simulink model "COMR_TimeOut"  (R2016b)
settings: Solver=FixedStepDiscrete  StartTime=0.0  StopTime=10.0  FixedStep=0.01  RelTol=1e-3  EnableMultiTasking=on
undefined symbols (not defined in the file or in its folder): bin2dec, COMR_cntObcTmtDiag_CW, COMR_cntVcu2A3TmtDiag_CW, COMR_flgTmtCAB_C, COMR_numPackVcuMsg_C, COMR_tiBusoffDiagEna_C, COMR_tiCabMsgTmt_C, COMR_tiCSCMsgTmt_C, COMR_tiGWMsg050Tmt_C, COMR_tiGWMsgTmt_C, COMR_tiHv638MsgTmt_C, COMR_tiMcuMsgTmt_C, COMR_tiObcMsgTmt_C, COMR_tiPackVcuMsgTmt_C, COMR_tiPwrupDiagEna_C, COMR_tiTmtBase_C, COMR_tiVcuMsgTmt_C, COMR_UAESFltDiagDisbl_C
libraries: simulink x167
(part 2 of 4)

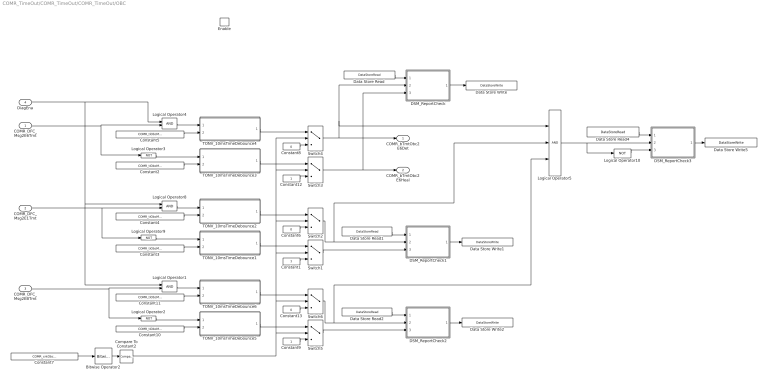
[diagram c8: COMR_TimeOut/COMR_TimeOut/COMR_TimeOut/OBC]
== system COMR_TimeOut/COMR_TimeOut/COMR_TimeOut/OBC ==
  COMR_DFC_Msg2E6Tmt : Inport
  COMR_DFC_Msg2E1Tmt : Inport  Port=2
  COMR_DFC_Msg2EBTmt : Inport  Port=3
  DiagEna : Inport  Port=4
  Enable : EnablePort
  Bitwise Operator2 : simulink/Logic and Bit Operations/Bitwise Operator  logicop=AND  UseBitMask=on  BitMask=bin2dec('00010000')  BitMaskRealWorld=Stored Integer
  Compare To Constant2 : simulink/Logic and Bit Operations/Compare To Constant  relop===  const=16  OutDataTypeStr=boolean
  Constant1 : Constant  OutDataTypeStr=boolean
  Constant{2..5,10..11} (6 alike) : Constant  Value=COMR_tiObcMsgTmt_C
  Constant12 : Constant  OutDataTypeStr=boolean
  Constant13 : Constant  Value=0  OutDataTypeStr=boolean
  Constant6 : Constant  Value=0  OutDataTypeStr=boolean
  Constant7 : Constant  Value=COMR_cntObcTmtDiag_CW
  Constant8 : Constant  Value=0  OutDataTypeStr=boolean
  Constant9 : Constant  OutDataTypeStr=boolean
  DSM_ReportCheck : Subsystem  TreatAsAtomicUnit=on  RTWFcnName=DSM_ReportCheck  RTWFileName=SrvLib
  DSM_ReportCheck1 : Subsystem  TreatAsAtomicUnit=on  RTWFcnName=DSM_ReportCheck  RTWFileName=SrvLib
  DSM_ReportCheck2 : Subsystem  TreatAsAtomicUnit=on  RTWFcnName=DSM_ReportCheck  RTWFileName=SrvLib
  DSM_ReportCheck3 : Subsystem  TreatAsAtomicUnit=on  RTWFcnName=DSM_ReportCheck  RTWFileName=SrvLib
  Data Store Read : DataStoreRead  DataStoreName=DFC_Msg2E6Tmt
  Data Store Read1 : DataStoreRead  DataStoreName=DFC_Msg2E1Tmt
  Data Store Read2 : DataStoreRead  DataStoreName=DFC_Msg2EBTmt
  Data Store Read4 : DataStoreRead  DataStoreName=DFC_ObcTmt
  Data Store Write : DataStoreWrite  DataStoreName=DFC_Msg2E6Tmt
  Data Store Write1 : DataStoreWrite  DataStoreName=DFC_Msg2E1Tmt
  Data Store Write2 : DataStoreWrite  DataStoreName=DFC_Msg2EBTmt
  Data Store Write5 : DataStoreWrite  DataStoreName=DFC_ObcTmt
  Logical Operator1 : Logic  AllPortsSameDT=off  OutDataTypeStr=boolean
  Logical Operator{2..3,9..10} (4 alike) : Logic  Operator=NOT  AllPortsSameDT=off  OutDataTypeStr=boolean
  Logical Operator4 : Logic  AllPortsSameDT=off  OutDataTypeStr=boolean
  Logical Operator5 : Logic  Inputs=3  AllPortsSameDT=off  OutDataTypeStr=boolean
  Logical Operator8 : Logic  AllPortsSameDT=off  OutDataTypeStr=boolean
  Switch{1..6} (6 alike) : Switch  Criteria=u2 > Threshold
  TONV_10msTimeDebounce1 : Subsystem  TreatAsAtomicUnit=on  RTWFcnName=TONV_10msTimeDebounce  RTWFileName=SrvLib
  TONV_10msTimeDebounce2 : Subsystem  TreatAsAtomicUnit=on  RTWFcnName=TONV_10msTimeDebounce  RTWFileName=SrvLib
  TONV_10msTimeDebounce3 : Subsystem  TreatAsAtomicUnit=on  RTWFcnName=TONV_10msTimeDebounce  RTWFileName=SrvLib
  TONV_10msTimeDebounce4 : Subsystem  TreatAsAtomicUnit=on  RTWFcnName=TONV_10msTimeDebounce  RTWFileName=SrvLib
  TONV_10msTimeDebounce5 : Subsystem  TreatAsAtomicUnit=on  RTWFcnName=TONV_10msTimeDebounce  RTWFileName=SrvLib
  TONV_10msTimeDebounce6 : Subsystem  TreatAsAtomicUnit=on  RTWFcnName=TONV_10msTimeDebounce  RTWFileName=SrvLib
  COMR_bTmtObc2E6Det : Outport  OutputWhenDisabled=reset  InitialOutput=[0]
  COMR_bTmtObc2E6Heal : Outport  Port=2  OutputWhenDisabled=reset  InitialOutput=[0]
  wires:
  Constant5/1 -> TONV_10msTimeDebounce4/2(T)
  DSM_ReportCheck/1(Dfc_id) -> Data Store Write/1
  Constant2/1 -> TONV_10msTimeDebounce3/2(T)
  Constant8/1 -> Switch4/3
  Constant12/1 -> Switch3/3
  TONV_10msTimeDebounce4/1(y) -> Switch4/1
  TONV_10msTimeDebounce3/1(y) -> Switch3/1
  Switch3/1 -> DSM_ReportCheck/3(Heal), COMR_bTmtObc2E6Heal/1
  Data Store Read/1 -> DSM_ReportCheck/1(Dfc_id_nv)
  Logical Operator3/1 -> TONV_10msTimeDebounce3/1(u)
  Switch4/1 -> DSM_ReportCheck/2(Err), Logical Operator5/1, COMR_bTmtObc2E6Det/1
  COMR_DFC_Msg2E6Tmt/1 -> Logical Operator3/1, Logical Operator4/2
  Logical Operator4/1 -> TONV_10msTimeDebounce4/1(u)
  Constant4/1 -> TONV_10msTimeDebounce2/2(T)
  DSM_ReportCheck1/1(Dfc_id) -> Data Store Write1/1
  Constant3/1 -> TONV_10msTimeDebounce1/2(T)
  Compare To Constant2/1 -> Switch5/2, Switch6/2, Switch3/2, Switch4/2, Switch2/2, Switch1/2
  Constant7/1 -> Bitwise Operator2/1
  Bitwise Operator2/1 -> Compare To Constant2/1
  Constant6/1 -> Switch2/3
  Constant1/1 -> Switch1/3
  TONV_10msTimeDebounce2/1(y) -> Switch2/1
  TONV_10msTimeDebounce1/1(y) -> Switch1/1
  Switch1/1 -> DSM_ReportCheck1/3(Heal)
  Data Store Read1/1 -> DSM_ReportCheck1/1(Dfc_id_nv)
  Switch2/1 -> DSM_ReportCheck1/2(Err), Logical Operator5/2
  COMR_DFC_Msg2E1Tmt/1 -> Logical Operator9/1, Logical Operator8/2
  Logical Operator8/1 -> TONV_10msTimeDebounce2/1(u)
  Logical Operator9/1 -> TONV_10msTimeDebounce1/1(u)
  DiagEna/1 -> Logical Operator1/1, Logical Operator8/1, Logical Operator4/1
  Constant11/1 -> TONV_10msTimeDebounce6/2(T)
  DSM_ReportCheck2/1(Dfc_id) -> Data Store Write2/1
  Constant10/1 -> TONV_10msTimeDebounce5/2(T)
  Constant13/1 -> Switch6/3
  Constant9/1 -> Switch5/3
  TONV_10msTimeDebounce6/1(y) -> Switch6/1
  TONV_10msTimeDebounce5/1(y) -> Switch5/1
  Switch5/1 -> DSM_ReportCheck2/3(Heal)
  Data Store Read2/1 -> DSM_ReportCheck2/1(Dfc_id_nv)
  Switch6/1 -> DSM_ReportCheck2/2(Err), Logical Operator5/3
  COMR_DFC_Msg2EBTmt/1 -> Logical Operator2/1, Logical Operator1/2
  Logical Operator1/1 -> TONV_10msTimeDebounce6/1(u)
  Logical Operator2/1 -> TONV_10msTimeDebounce5/1(u)
  Data Store Read4/1 -> DSM_ReportCheck3/1(Dfc_id_nv)
  DSM_ReportCheck3/1(Dfc_id) -> Data Store Write5/1
  Logical Operator5/1 -> DSM_ReportCheck3/2(Err), Logical Operator10/1
  Logical Operator10/1 -> DSM_ReportCheck3/3(Heal)

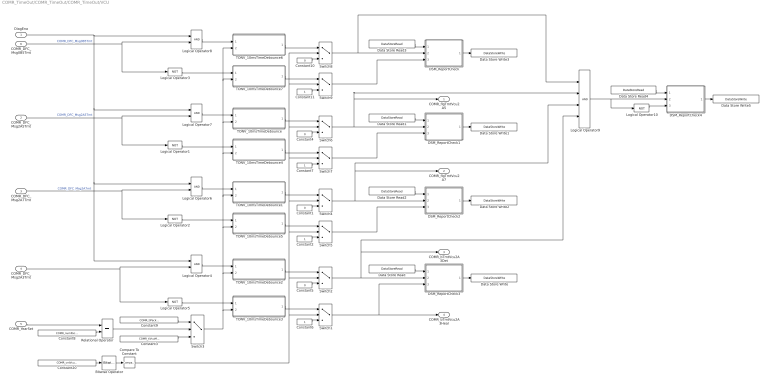
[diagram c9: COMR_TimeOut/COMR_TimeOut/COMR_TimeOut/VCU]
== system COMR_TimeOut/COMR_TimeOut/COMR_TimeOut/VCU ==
  DiagEna : Inport
  COMR_DFC_Msg2A5Tmt : Inport  Port=2
  COMR_DFC_Msg2A7Tmt : Inport  Port=3
  COMR_DFC_Msg2A3Tmt : Inport  Port=4
  COMR_YearSet : Inport  Port=5
  COMR_DFC_Msg0B5Tmt : Inport  Port=6
  Bitwise Operator : simulink/Logic and Bit Operations/Bitwise Operator  logicop=AND  UseBitMask=on  BitMask=bin2dec('00010000')  BitMaskRealWorld=Stored Integer
  Compare To Constant : simulink/Logic and Bit Operations/Compare To Constant  relop===  const=16  OutDataTypeStr=boolean
  Constant{1,4..5,10} (4 alike) : Constant  Value=0  OutDataTypeStr=boolean
  Constant{2,6..7,11} (4 alike) : Constant  OutDataTypeStr=boolean
  Constant20 : Constant  Value=COMR_cntVcu2A3TmtDiag_CW
  Constant3 : Constant  Value=COMR_tiVcuMsgTmt_C
  Constant8 : Constant  Value=COMR_numPackVcuMsg_C  OutDataTypeStr=uint16
  Constant9 : Constant  Value=COMR_tiPackVcuMsgTmt_C
  DSM_ReportCheck : Subsystem  TreatAsAtomicUnit=on  RTWFcnName=DSM_ReportCheck  RTWFileName=SrvLib
  DSM_ReportCheck1 : Subsystem  TreatAsAtomicUnit=on  RTWFcnName=DSM_ReportCheck  RTWFileName=SrvLib
  DSM_ReportCheck2 : Subsystem  TreatAsAtomicUnit=on  RTWFcnName=DSM_ReportCheck  RTWFileName=SrvLib
  DSM_ReportCheck3 : Subsystem  TreatAsAtomicUnit=on  RTWFcnName=DSM_ReportCheck  RTWFileName=SrvLib
  DSM_ReportCheck4 : Subsystem  TreatAsAtomicUnit=on  RTWFcnName=DSM_ReportCheck  RTWFileName=SrvLib
  Data Store Read : DataStoreRead  DataStoreName=DFC_Msg2A3Tmt
  Data Store Read1 : DataStoreRead  DataStoreName=DFC_Msg2A5Tmt
  Data Store Read2 : DataStoreRead  DataStoreName=DFC_Msg2A7Tmt
  Data Store Read3 : DataStoreRead  DataStoreName=DFC_Msg0B5Tmt
  Data Store Read4 : DataStoreRead  DataStoreName=DFC_VcuTmt
  Data Store Write : DataStoreWrite  DataStoreName=DFC_Msg2A3Tmt
  Data Store Write1 : DataStoreWrite  DataStoreName=DFC_Msg2A5Tmt
  Data Store Write2 : DataStoreWrite  DataStoreName=DFC_Msg2A7Tmt
  Data Store Write3 : DataStoreWrite  DataStoreName=DFC_Msg0B5Tmt
  Data Store Write5 : DataStoreWrite  DataStoreName=DFC_VcuTmt
  Logical Operator{1..3,5,10} (5 alike) : Logic  Operator=NOT  AllPortsSameDT=off  OutDataTypeStr=boolean
  Logical Operator{4,6..8} (4 alike) : Logic  AllPortsSameDT=off  OutDataTypeStr=boolean
  Logical Operator9 : Logic  Inputs=4  AllPortsSameDT=off  OutDataTypeStr=boolean
  Relational Operator : RelationalOperator  Operator===  OutDataTypeStr=boolean  RndMeth=Simplest
  Switch{1..2,4..9} (8 alike) : Switch  Criteria=u2 > Threshold
  Switch3 : Switch  Criteria=u2 ~= 0
  TONV_10msTimeDebounce : Subsystem  TreatAsAtomicUnit=on  RTWFcnName=TONV_10msTimeDebounce  RTWFileName=SrvLib
  TONV_10msTimeDebounce1 : Subsystem  TreatAsAtomicUnit=on  RTWFcnName=TONV_10msTimeDebounce  RTWFileName=SrvLib
  TONV_10msTimeDebounce2 : Subsystem  TreatAsAtomicUnit=on  RTWFcnName=TONV_10msTimeDebounce  RTWFileName=SrvLib
  TONV_10msTimeDebounce3 : Subsystem  TreatAsAtomicUnit=on  RTWFcnName=TONV_10msTimeDebounce  RTWFileName=SrvLib
  TONV_10msTimeDebounce4 : Subsystem  TreatAsAtomicUnit=on  RTWFcnName=TONV_10msTimeDebounce  RTWFileName=SrvLib
  TONV_10msTimeDebounce5 : Subsystem  TreatAsAtomicUnit=on  RTWFcnName=TONV_10msTimeDebounce  RTWFileName=SrvLib
  TONV_10msTimeDebounce6 : Subsystem  TreatAsAtomicUnit=on  RTWFcnName=TONV_10msTimeDebounce  RTWFileName=SrvLib
  TONV_10msTimeDebounce7 : Subsystem  TreatAsAtomicUnit=on  RTWFcnName=TONV_10msTimeDebounce  RTWFileName=SrvLib
  COMR_flgTmtVcu2A5 : Outport
  COMR_flgTmtVcu2A7 : Outport  Port=2
  COMR_bTmtVcu2A3Det : Outport  Port=3  OutputWhenDisabled=reset  InitialOutput=[0]
  COMR_bTmtVcu2A3Heal : Outport  Port=4  OutputWhenDisabled=reset  InitialOutput=[0]
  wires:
  COMR_DFC_Msg2A5Tmt/1 -> Logical Operator7/2, Logical Operator1/1  "COMR_DFC_Msg2A5Tmt"
  COMR_DFC_Msg2A7Tmt/1 -> Logical Operator6/2, Logical Operator2/1  "COMR_DFC_Msg2A7mt"
  Constant3/1 -> Switch3/3
  TONV_10msTimeDebounce2/1(y) -> Switch2/1
  Constant20/1 -> Bitwise Operator/1
  Bitwise Operator/1 -> Compare To Constant/1
  Constant5/1 -> Switch2/3
  Constant6/1 -> Switch1/3
  TONV_10msTimeDebounce3/1(y) -> Switch1/1
  Switch2/1 -> DSM_ReportCheck3/2(Err), Logical Operator9/4, COMR_bTmtVcu2A3Det/1
  Switch1/1 -> DSM_ReportCheck3/3(Heal), COMR_bTmtVcu2A3Heal/1
  DSM_ReportCheck3/1(Dfc_id) -> Data Store Write/1
  Data Store Read/1 -> DSM_ReportCheck3/1(Dfc_id_nv)
  COMR_DFC_Msg2A3Tmt/1 -> Logical Operator4/2, Logical Operator5/1
  Logical Operator4/1 -> TONV_10msTimeDebounce2/1(u)
  DiagEna/1 -> Logical Operator8/1, Logical Operator7/1, Logical Operator4/1, Logical Operator6/1
  COMR_YearSet/1 -> Relational Operator/1
  Relational Operator/1 -> Switch3/2
  Constant8/1 -> Relational Operator/2
  Constant9/1 -> Switch3/1
  Logical Operator5/1 -> TONV_10msTimeDebounce3/1(u)
  Data Store Read1/1 -> DSM_ReportCheck1/1(Dfc_id_nv)
  Switch6/1 -> DSM_ReportCheck1/2(Err), Logical Operator9/2, COMR_flgTmtVcu2A5/1
  DSM_ReportCheck1/1(Dfc_id) -> Data Store Write1/1
  Logical Operator1/1 -> TONV_10msTimeDebounce4/1(u)
  Switch7/1 -> DSM_ReportCheck1/3(Heal)
  Switch3/1 -> TONV_10msTimeDebounce3/2(T), TONV_10msTimeDebounce2/2(T), TONV_10msTimeDebounce6/2(T), TONV_10msTimeDebounce7/2(T), TONV_10msTimeDebounce/2(T), TONV_10msTimeDebounce4/2(T), TONV_10msTimeDebounce1/2(T), TONV_10msTimeDebounce5/2(T)
  Logical Operator2/1 -> TONV_10msTimeDebounce5/1(u)
  Data Store Read2/1 -> DSM_ReportCheck2/1(Dfc_id_nv)
  Switch4/1 -> DSM_ReportCheck2/2(Err), COMR_flgTmtVcu2A7/1, Logical Operator9/3
  DSM_ReportCheck2/1(Dfc_id) -> Data Store Write2/1
  COMR_DFC_Msg0B5Tmt/1 -> Logical Operator8/2, Logical Operator3/1  "COMR_DFC_Msg0B5Tmt"
  Data Store Read3/1 -> DSM_ReportCheck/1(Dfc_id_nv)
  Switch8/1 -> DSM_ReportCheck/2(Err), Logical Operator9/1
  DSM_ReportCheck/1(Dfc_id) -> Data Store Write3/1
  Logical Operator3/1 -> TONV_10msTimeDebounce7/1(u)
  Switch9/1 -> DSM_ReportCheck/3(Heal)
  TONV_10msTimeDebounce1/1(y) -> Switch4/1
  Constant1/1 -> Switch4/3
  TONV_10msTimeDebounce5/1(y) -> Switch5/1
  Constant2/1 -> Switch5/3
  Switch5/1 -> DSM_ReportCheck2/3(Heal)
  Constant4/1 -> Switch6/3
  Constant7/1 -> Switch7/3
  TONV_10msTimeDebounce/1(y) -> Switch6/1
  TONV_10msTimeDebounce4/1(y) -> Switch7/1
  Constant10/1 -> Switch8/3
  Constant11/1 -> Switch9/3
  Compare To Constant/1 -> Switch2/2, Switch5/2, Switch7/2, Switch9/2, Switch8/2, Switch6/2, Switch4/2, Switch1/2
  TONV_10msTimeDebounce6/1(y) -> Switch8/1
  TONV_10msTimeDebounce7/1(y) -> Switch9/1
  Logical Operator6/1 -> TONV_10msTimeDebounce1/1(u)
  Logical Operator7/1 -> TONV_10msTimeDebounce/1(u)
  Logical Operator8/1 -> TONV_10msTimeDebounce6/1(u)
  Data Store Read4/1 -> DSM_ReportCheck4/1(Dfc_id_nv)
  DSM_ReportCheck4/1(Dfc_id) -> Data Store Write5/1
  Logical Operator9/1 -> DSM_ReportCheck4/2(Err), Logical Operator10/1
  Logical Operator10/1 -> DSM_ReportCheck4/3(Heal)

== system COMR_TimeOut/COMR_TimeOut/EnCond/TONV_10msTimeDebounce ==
  note: Turn On Delay Time Deboune
  u : Inport
  T : Inport  Port=2
  Add : Sum
  Constant1 : Constant  Value=0  OutDataTypeStr=single
  Constant2 : Constant  OutDataTypeStr=uint8
  Constant3 : Constant  Value=0  OutDataTypeStr=uint8
  Constant4 : Constant  Value=0.01  OutDataTypeStr=single
  Delay : Delay  DelayLength=1  InitialCondition=0
  MinMax : MinMax  Inputs=2
  Product : Product  OutMin=[0]  OutMax=[65535]  OutDataTypeStr=single
  Relational Operator : RelationalOperator  Operator=>  OutDataTypeStr=boolean  RndMeth=Simplest
  Switch : Switch  Criteria=u2 ~= 0
  Switch1 : Switch  Criteria=u2 ~= 0
  y : Outport
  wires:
  MinMax/1 -> Add/2
  T/1 -> Relational Operator/2, MinMax/1
  Relational Operator/1 -> y/1
  Delay/1 -> MinMax/2
  Switch/1 -> Add/1
  Product/1 -> Delay/1, Relational Operator/1
  Add/1 -> Product/2
  Constant1/1 -> Switch/3
  Constant4/1 -> Switch/1
  u/1 -> Switch/2, Switch1/2
  Constant2/1 -> Switch1/1
  Constant3/1 -> Switch1/3
  Switch1/1 -> Product/1

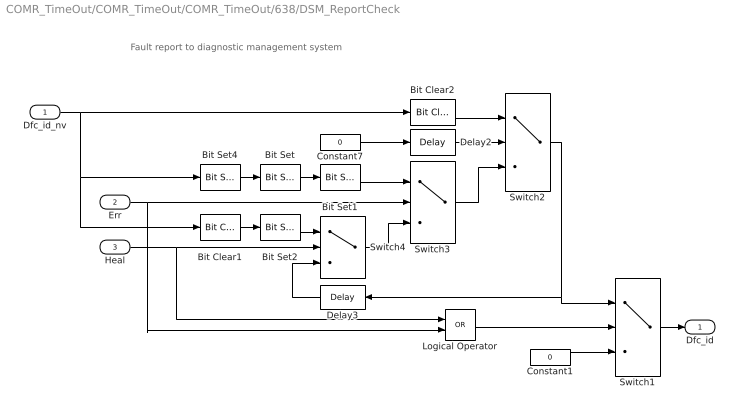
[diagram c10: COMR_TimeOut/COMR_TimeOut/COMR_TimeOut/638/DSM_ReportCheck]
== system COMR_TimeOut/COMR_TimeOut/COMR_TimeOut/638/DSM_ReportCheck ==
  note: Fault report to diagnostic management system
  Dfc_id_nv : Inport  OutDataTypeStr=uint8
  Err : Inport  Port=2
  Heal : Inport  Port=3
  Bit Clear1 : simulink/Logic and Bit Operations/Bit Clear  iBit=4
  Bit Clear2 : simulink/Logic and Bit Operations/Bit Clear  iBit=3
  Bit Set : simulink/Logic and Bit Operations/Bit Set  iBit=4
  Bit Set1 : simulink/Logic and Bit Operations/Bit Set  iBit=3
  Bit Set2 : simulink/Logic and Bit Operations/Bit Set  iBit=3
  Bit Set4 : simulink/Logic and Bit Operations/Bit Set  iBit=7
  Constant1 : Constant  Value=0  OutDataTypeStr=uint8
  Constant7 : Constant  Value=0  OutDataTypeStr=boolean
  Delay2 : Delay  DelayLength=1  InitialCondition=1
  Delay3 : Delay  DelayLength=1  InitialCondition=0
  Logical Operator : Logic  Operator=OR  AllPortsSameDT=off  OutDataTypeStr=boolean
  Switch{1..4} (4 alike) : Switch  Criteria=u2 ~= 0
  Dfc_id : Outport  OutDataTypeStr=uint8
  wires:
  Dfc_id_nv/1 -> Bit Clear2/1, Bit Set4/1, Bit Clear1/1
  Bit Set4/1 -> Bit Set/1
  Constant7/1 -> Delay2/1
  Delay2/1 -> Switch2/2
  Switch3/1 -> Switch2/3
  Bit Clear2/1 -> Switch2/1
  Switch2/1 -> Delay3/1, Switch1/1
  Bit Set1/1 -> Switch3/1
  Bit Set/1 -> Bit Set1/1
  Switch4/1 -> Switch3/3
  Err/1 -> Logical Operator/2, Switch3/2
  Bit Set2/1 -> Switch4/1
  Bit Clear1/1 -> Bit Set2/1
  Delay3/1 -> Switch4/3
  Heal/1 -> Logical Operator/1, Switch4/2
  Logical Operator/1 -> Switch1/2
  Constant1/1 -> Switch1/3
  Switch1/1 -> Dfc_id/1

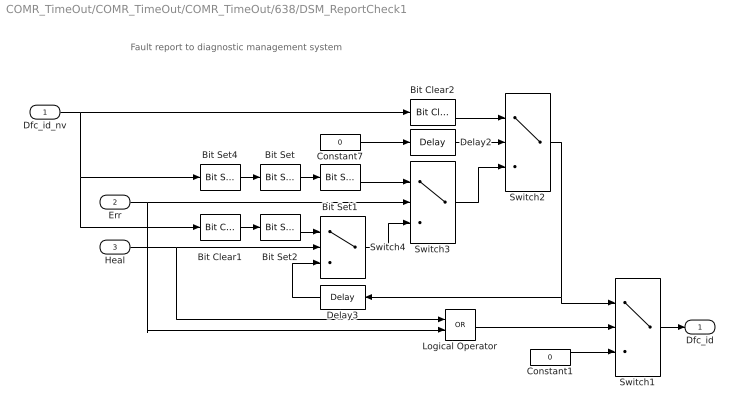
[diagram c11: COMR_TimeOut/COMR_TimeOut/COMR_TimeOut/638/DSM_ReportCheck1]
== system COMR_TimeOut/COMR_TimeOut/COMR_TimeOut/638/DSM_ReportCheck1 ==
  note: Fault report to diagnostic management system
  Dfc_id_nv : Inport  OutDataTypeStr=uint8
  Err : Inport  Port=2
  Heal : Inport  Port=3
  Bit Clear1 : simulink/Logic and Bit Operations/Bit Clear  iBit=4
  Bit Clear2 : simulink/Logic and Bit Operations/Bit Clear  iBit=3
  Bit Set : simulink/Logic and Bit Operations/Bit Set  iBit=4
  Bit Set1 : simulink/Logic and Bit Operations/Bit Set  iBit=3
  Bit Set2 : simulink/Logic and Bit Operations/Bit Set  iBit=3
  Bit Set4 : simulink/Logic and Bit Operations/Bit Set  iBit=7
  Constant1 : Constant  Value=0  OutDataTypeStr=uint8
  Constant7 : Constant  Value=0  OutDataTypeStr=boolean
  Delay2 : Delay  DelayLength=1  InitialCondition=1
  Delay3 : Delay  DelayLength=1  InitialCondition=0
  Logical Operator : Logic  Operator=OR  AllPortsSameDT=off  OutDataTypeStr=boolean
  Switch{1..4} (4 alike) : Switch  Criteria=u2 ~= 0
  Dfc_id : Outport  OutDataTypeStr=uint8
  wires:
  Switch1/1 -> Dfc_id/1
  Constant1/1 -> Switch1/3
  Logical Operator/1 -> Switch1/2
  Heal/1 -> Switch4/2, Logical Operator/1
  Delay3/1 -> Switch4/3
  Bit Clear1/1 -> Bit Set2/1
  Bit Set2/1 -> Switch4/1
  Err/1 -> Switch3/2, Logical Operator/2
  Switch4/1 -> Switch3/3
  Bit Set/1 -> Bit Set1/1
  Bit Set1/1 -> Switch3/1
  Switch2/1 -> Switch1/1, Delay3/1
  Bit Clear2/1 -> Switch2/1
  Switch3/1 -> Switch2/3
  Delay2/1 -> Switch2/2
  Constant7/1 -> Delay2/1
  Bit Set4/1 -> Bit Set/1
  Dfc_id_nv/1 -> Bit Clear1/1, Bit Set4/1, Bit Clear2/1

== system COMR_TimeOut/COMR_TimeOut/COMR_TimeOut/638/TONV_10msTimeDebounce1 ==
  note: Turn On Delay Time Deboune
  u : Inport
  T : Inport  Port=2
  Add : Sum
  Constant1 : Constant  Value=0  OutDataTypeStr=single
  Constant2 : Constant  OutDataTypeStr=uint8
  Constant3 : Constant  Value=0  OutDataTypeStr=uint8
  Constant4 : Constant  Value=0.01  OutDataTypeStr=single
  Delay : Delay  DelayLength=1  InitialCondition=0
  MinMax : MinMax  Inputs=2
  Product : Product  OutMin=[0]  OutMax=[65535]  OutDataTypeStr=single
  Relational Operator : RelationalOperator  Operator=>  OutDataTypeStr=boolean  RndMeth=Simplest
  Switch : Switch  Criteria=u2 ~= 0
  Switch1 : Switch  Criteria=u2 ~= 0
  y : Outport
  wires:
  MinMax/1 -> Add/2
  T/1 -> Relational Operator/2, MinMax/1
  Relational Operator/1 -> y/1
  Delay/1 -> MinMax/2
  Switch/1 -> Add/1
  Product/1 -> Delay/1, Relational Operator/1
  Add/1 -> Product/2
  Constant1/1 -> Switch/3
  Constant4/1 -> Switch/1
  u/1 -> Switch/2, Switch1/2
  Constant2/1 -> Switch1/1
  Constant3/1 -> Switch1/3
  Switch1/1 -> Product/1

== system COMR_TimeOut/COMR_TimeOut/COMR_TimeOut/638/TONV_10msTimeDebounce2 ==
  note: Turn On Delay Time Deboune
  u : Inport
  T : Inport  Port=2
  Add : Sum
  Constant1 : Constant  Value=0  OutDataTypeStr=single
  Constant2 : Constant  OutDataTypeStr=uint8
  Constant3 : Constant  Value=0  OutDataTypeStr=uint8
  Constant4 : Constant  Value=0.01  OutDataTypeStr=single
  Delay : Delay  DelayLength=1  InitialCondition=0
  MinMax : MinMax  Inputs=2
  Product : Product  OutMin=[0]  OutMax=[65535]  OutDataTypeStr=single
  Relational Operator : RelationalOperator  Operator=>  OutDataTypeStr=boolean  RndMeth=Simplest
  Switch : Switch  Criteria=u2 ~= 0
  Switch1 : Switch  Criteria=u2 ~= 0
  y : Outport
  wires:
  MinMax/1 -> Add/2
  T/1 -> Relational Operator/2, MinMax/1
  Relational Operator/1 -> y/1
  Delay/1 -> MinMax/2
  Switch/1 -> Add/1
  Product/1 -> Delay/1, Relational Operator/1
  Add/1 -> Product/2
  Constant1/1 -> Switch/3
  Constant4/1 -> Switch/1
  u/1 -> Switch/2, Switch1/2
  Constant2/1 -> Switch1/1
  Constant3/1 -> Switch1/3
  Switch1/1 -> Product/1

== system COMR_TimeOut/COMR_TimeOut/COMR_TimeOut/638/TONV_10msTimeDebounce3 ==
  note: Turn On Delay Time Deboune
  u : Inport
  T : Inport  Port=2
  Add : Sum
  Constant1 : Constant  Value=0  OutDataTypeStr=single
  Constant2 : Constant  OutDataTypeStr=uint8
  Constant3 : Constant  Value=0  OutDataTypeStr=uint8
  Constant4 : Constant  Value=0.01  OutDataTypeStr=single
  Delay : Delay  DelayLength=1  InitialCondition=0
  MinMax : MinMax  Inputs=2
  Product : Product  OutMin=[0]  OutMax=[65535]  OutDataTypeStr=single
  Relational Operator : RelationalOperator  Operator=>  OutDataTypeStr=boolean  RndMeth=Simplest
  Switch : Switch  Criteria=u2 ~= 0
  Switch1 : Switch  Criteria=u2 ~= 0
  y : Outport
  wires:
  MinMax/1 -> Add/2
  T/1 -> Relational Operator/2, MinMax/1
  Relational Operator/1 -> y/1
  Delay/1 -> MinMax/2
  Switch/1 -> Add/1
  Product/1 -> Delay/1, Relational Operator/1
  Add/1 -> Product/2
  Constant1/1 -> Switch/3
  Constant4/1 -> Switch/1
  u/1 -> Switch/2, Switch1/2
  Constant2/1 -> Switch1/1
  Constant3/1 -> Switch1/3
  Switch1/1 -> Product/1

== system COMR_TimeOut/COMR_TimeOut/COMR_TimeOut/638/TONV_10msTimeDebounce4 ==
  note: Turn On Delay Time Deboune
  u : Inport
  T : Inport  Port=2
  Add : Sum
  Constant1 : Constant  Value=0  OutDataTypeStr=single
  Constant2 : Constant  OutDataTypeStr=uint8
  Constant3 : Constant  Value=0  OutDataTypeStr=uint8
  Constant4 : Constant  Value=0.01  OutDataTypeStr=single
  Delay : Delay  DelayLength=1  InitialCondition=0
  MinMax : MinMax  Inputs=2
  Product : Product  OutMin=[0]  OutMax=[65535]  OutDataTypeStr=single
  Relational Operator : RelationalOperator  Operator=>  OutDataTypeStr=boolean  RndMeth=Simplest
  Switch : Switch  Criteria=u2 ~= 0
  Switch1 : Switch  Criteria=u2 ~= 0
  y : Outport
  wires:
  MinMax/1 -> Add/2
  T/1 -> Relational Operator/2, MinMax/1
  Relational Operator/1 -> y/1
  Delay/1 -> MinMax/2
  Switch/1 -> Add/1
  Product/1 -> Delay/1, Relational Operator/1
  Add/1 -> Product/2
  Constant1/1 -> Switch/3
  Constant4/1 -> Switch/1
  u/1 -> Switch/2, Switch1/2
  Constant2/1 -> Switch1/1
  Constant3/1 -> Switch1/3
  Switch1/1 -> Product/1

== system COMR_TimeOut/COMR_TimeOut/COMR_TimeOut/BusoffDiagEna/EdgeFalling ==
  u : Inport
  Delay1 : Delay  DelayLength=1  InitialCondition=0
  Logical Operator3 : Logic  Operator=NOT  AllPortsSameDT=off  OutDataTypeStr=boolean
  Logical Operator4 : Logic  AllPortsSameDT=off  OutDataTypeStr=boolean
  y : Outport
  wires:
  Delay1/1 -> Logical Operator4/1
  Logical Operator3/1 -> Logical Operator4/2
  u/1 -> Logical Operator3/1, Delay1/1
  Logical Operator4/1 -> y/1

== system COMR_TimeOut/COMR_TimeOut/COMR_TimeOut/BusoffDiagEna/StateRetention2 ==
  u : Inport
  clc : Inport  Port=2
  Constant1 : Constant  Value=COMR_tiTmtBase_C
  Constant2 : Constant  Value=COMR_tiBusoffDiagEna_C
  Constant8 : Constant  Value=single(0)
  Delay2 : Delay  DelayLength=1  InitialCondition=0
  EdgeRising : Subsystem  TreatAsAtomicUnit=on  RTWFcnName=EdgeRising  RTWFileName=SrvLib
  Logical Operator : Logic  Operator=OR  AllPortsSameDT=off  OutDataTypeStr=boolean
  Relational Operator2 : RelationalOperator  Operator=>  OutDataTypeStr=boolean  RndMeth=Simplest
  Subsystem3 : Subsystem
  Timer : Subsystem
  _Out : Outport
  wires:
  Subsystem3/1(Q) -> Timer/1(En)
  Delay2/1 -> EdgeRising/1(u), Logical Operator/2
  Constant2/1 -> Relational Operator2/2
  Constant8/1 -> Timer/4(Vst)
  Timer/1(Timer) -> Relational Operator2/1
  EdgeRising/1(y) -> Timer/3(Rst)
  Constant1/1 -> Timer/2(Ts)
  Relational Operator2/1 -> Delay2/1
  u/1 -> Subsystem3/1(set)
  Logical Operator/1 -> Subsystem3/2(clear)
  clc/1 -> Logical Operator/1
  Subsystem3/2(_Q) -> _Out/1

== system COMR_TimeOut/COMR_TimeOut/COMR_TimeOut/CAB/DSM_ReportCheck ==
  note: Fault report to diagnostic management system
  Dfc_id_nv : Inport  OutDataTypeStr=uint8
  Err : Inport  Port=2
  Heal : Inport  Port=3
  Bit Clear1 : simulink/Logic and Bit Operations/Bit Clear  iBit=4
  Bit Clear2 : simulink/Logic and Bit Operations/Bit Clear  iBit=3
  Bit Set : simulink/Logic and Bit Operations/Bit Set  iBit=4
  Bit Set1 : simulink/Logic and Bit Operations/Bit Set  iBit=3
  Bit Set2 : simulink/Logic and Bit Operations/Bit Set  iBit=3
  Bit Set4 : simulink/Logic and Bit Operations/Bit Set  iBit=7
  Constant1 : Constant  Value=0  OutDataTypeStr=uint8
  Constant7 : Constant  Value=0  OutDataTypeStr=boolean
  Delay2 : Delay  DelayLength=1  InitialCondition=1
  Delay3 : Delay  DelayLength=1  InitialCondition=0
  Logical Operator : Logic  Operator=OR  AllPortsSameDT=off  OutDataTypeStr=boolean
  Switch{1..4} (4 alike) : Switch  Criteria=u2 ~= 0
  Dfc_id : Outport  OutDataTypeStr=uint8
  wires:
  Dfc_id_nv/1 -> Bit Clear2/1, Bit Set4/1, Bit Clear1/1
  Bit Set4/1 -> Bit Set/1
  Constant7/1 -> Delay2/1
  Delay2/1 -> Switch2/2
  Switch3/1 -> Switch2/3
  Bit Clear2/1 -> Switch2/1
  Switch2/1 -> Delay3/1, Switch1/1
  Bit Set1/1 -> Switch3/1
  Bit Set/1 -> Bit Set1/1
  Switch4/1 -> Switch3/3
  Err/1 -> Logical Operator/2, Switch3/2
  Bit Set2/1 -> Switch4/1
  Bit Clear1/1 -> Bit Set2/1
  Delay3/1 -> Switch4/3
  Heal/1 -> Logical Operator/1, Switch4/2
  Logical Operator/1 -> Switch1/2
  Constant1/1 -> Switch1/3
  Switch1/1 -> Dfc_id/1

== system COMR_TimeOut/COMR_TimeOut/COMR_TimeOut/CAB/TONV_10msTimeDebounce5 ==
  note: Turn On Delay Time Deboune
  u : Inport
  T : Inport  Port=2
  Add : Sum
  Constant1 : Constant  Value=0  OutDataTypeStr=single
  Constant2 : Constant  OutDataTypeStr=uint8
  Constant3 : Constant  Value=0  OutDataTypeStr=uint8
  Constant4 : Constant  Value=0.01  OutDataTypeStr=single
  Delay : Delay  DelayLength=1  InitialCondition=0
  MinMax : MinMax  Inputs=2
  Product : Product  OutMin=[0]  OutMax=[65535]  OutDataTypeStr=single
  Relational Operator : RelationalOperator  Operator=>  OutDataTypeStr=boolean  RndMeth=Simplest
  Switch : Switch  Criteria=u2 ~= 0
  Switch1 : Switch  Criteria=u2 ~= 0
  y : Outport
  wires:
  MinMax/1 -> Add/2
  T/1 -> Relational Operator/2, MinMax/1
  Relational Operator/1 -> y/1
  Delay/1 -> MinMax/2
  Switch/1 -> Add/1
  Product/1 -> Delay/1, Relational Operator/1
  Add/1 -> Product/2
  Constant1/1 -> Switch/3
  Constant4/1 -> Switch/1
  u/1 -> Switch/2, Switch1/2
  Constant2/1 -> Switch1/1
  Constant3/1 -> Switch1/3
  Switch1/1 -> Product/1

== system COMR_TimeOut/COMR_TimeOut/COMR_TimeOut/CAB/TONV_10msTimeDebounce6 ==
  note: Turn On Delay Time Deboune
  u : Inport
  T : Inport  Port=2
  Add : Sum
  Constant1 : Constant  Value=0  OutDataTypeStr=single
  Constant2 : Constant  OutDataTypeStr=uint8
  Constant3 : Constant  Value=0  OutDataTypeStr=uint8
  Constant4 : Constant  Value=0.01  OutDataTypeStr=single
  Delay : Delay  DelayLength=1  InitialCondition=0
  MinMax : MinMax  Inputs=2
  Product : Product  OutMin=[0]  OutMax=[65535]  OutDataTypeStr=single
  Relational Operator : RelationalOperator  Operator=>  OutDataTypeStr=boolean  RndMeth=Simplest
  Switch : Switch  Criteria=u2 ~= 0
  Switch1 : Switch  Criteria=u2 ~= 0
  y : Outport
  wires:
  MinMax/1 -> Add/2
  T/1 -> Relational Operator/2, MinMax/1
  Relational Operator/1 -> y/1
  Delay/1 -> MinMax/2
  Switch/1 -> Add/1
  Product/1 -> Delay/1, Relational Operator/1
  Add/1 -> Product/2
  Constant1/1 -> Switch/3
  Constant4/1 -> Switch/1
  u/1 -> Switch/2, Switch1/2
  Constant2/1 -> Switch1/1
  Constant3/1 -> Switch1/3
  Switch1/1 -> Product/1

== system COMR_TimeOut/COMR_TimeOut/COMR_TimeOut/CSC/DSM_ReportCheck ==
  note: Fault report to diagnostic management system
  Dfc_id_nv : Inport  OutDataTypeStr=uint8
  Err : Inport  Port=2
  Heal : Inport  Port=3
  Bit Clear1 : simulink/Logic and Bit Operations/Bit Clear  iBit=4
  Bit Clear2 : simulink/Logic and Bit Operations/Bit Clear  iBit=3
  Bit Set : simulink/Logic and Bit Operations/Bit Set  iBit=4
  Bit Set1 : simulink/Logic and Bit Operations/Bit Set  iBit=3
  Bit Set2 : simulink/Logic and Bit Operations/Bit Set  iBit=3
  Bit Set4 : simulink/Logic and Bit Operations/Bit Set  iBit=7
  Constant1 : Constant  Value=0  OutDataTypeStr=uint8
  Constant7 : Constant  Value=0  OutDataTypeStr=boolean
  Delay2 : Delay  DelayLength=1  InitialCondition=1
  Delay3 : Delay  DelayLength=1  InitialCondition=0
  Logical Operator : Logic  Operator=OR  AllPortsSameDT=off  OutDataTypeStr=boolean
  Switch{1..4} (4 alike) : Switch  Criteria=u2 ~= 0
  Dfc_id : Outport  OutDataTypeStr=uint8
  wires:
  Dfc_id_nv/1 -> Bit Clear2/1, Bit Set4/1, Bit Clear1/1
  Bit Set4/1 -> Bit Set/1
  Constant7/1 -> Delay2/1
  Delay2/1 -> Switch2/2
  Switch3/1 -> Switch2/3
  Bit Clear2/1 -> Switch2/1
  Switch2/1 -> Delay3/1, Switch1/1
  Bit Set1/1 -> Switch3/1
  Bit Set/1 -> Bit Set1/1
  Switch4/1 -> Switch3/3
  Err/1 -> Logical Operator/2, Switch3/2
  Bit Set2/1 -> Switch4/1
  Bit Clear1/1 -> Bit Set2/1
  Delay3/1 -> Switch4/3
  Heal/1 -> Logical Operator/1, Switch4/2
  Logical Operator/1 -> Switch1/2
  Constant1/1 -> Switch1/3
  Switch1/1 -> Dfc_id/1

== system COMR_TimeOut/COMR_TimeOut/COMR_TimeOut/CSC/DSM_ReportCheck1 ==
  note: Fault report to diagnostic management system
  Dfc_id_nv : Inport  OutDataTypeStr=uint8
  Err : Inport  Port=2
  Heal : Inport  Port=3
  Bit Clear1 : simulink/Logic and Bit Operations/Bit Clear  iBit=4
  Bit Clear2 : simulink/Logic and Bit Operations/Bit Clear  iBit=3
  Bit Set : simulink/Logic and Bit Operations/Bit Set  iBit=4
  Bit Set1 : simulink/Logic and Bit Operations/Bit Set  iBit=3
  Bit Set2 : simulink/Logic and Bit Operations/Bit Set  iBit=3
  Bit Set4 : simulink/Logic and Bit Operations/Bit Set  iBit=7
  Constant1 : Constant  Value=0  OutDataTypeStr=uint8
  Constant7 : Constant  Value=0  OutDataTypeStr=boolean
  Delay2 : Delay  DelayLength=1  InitialCondition=1
  Delay3 : Delay  DelayLength=1  InitialCondition=0
  Logical Operator : Logic  Operator=OR  AllPortsSameDT=off  OutDataTypeStr=boolean
  Switch{1..4} (4 alike) : Switch  Criteria=u2 ~= 0
  Dfc_id : Outport  OutDataTypeStr=uint8
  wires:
  Switch1/1 -> Dfc_id/1
  Constant1/1 -> Switch1/3
  Logical Operator/1 -> Switch1/2
  Heal/1 -> Switch4/2, Logical Operator/1
  Delay3/1 -> Switch4/3
  Bit Clear1/1 -> Bit Set2/1
  Bit Set2/1 -> Switch4/1
  Err/1 -> Switch3/2, Logical Operator/2
  Switch4/1 -> Switch3/3
  Bit Set/1 -> Bit Set1/1
  Bit Set1/1 -> Switch3/1
  Switch2/1 -> Switch1/1, Delay3/1
  Bit Clear2/1 -> Switch2/1
  Switch3/1 -> Switch2/3
  Delay2/1 -> Switch2/2
  Constant7/1 -> Delay2/1
  Bit Set4/1 -> Bit Set/1
  Dfc_id_nv/1 -> Bit Clear1/1, Bit Set4/1, Bit Clear2/1

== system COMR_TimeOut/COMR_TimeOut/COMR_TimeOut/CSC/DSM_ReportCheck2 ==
  note: Fault report to diagnostic management system
  Dfc_id_nv : Inport  OutDataTypeStr=uint8
  Err : Inport  Port=2
  Heal : Inport  Port=3
  Bit Clear1 : simulink/Logic and Bit Operations/Bit Clear  iBit=4
  Bit Clear2 : simulink/Logic and Bit Operations/Bit Clear  iBit=3
  Bit Set : simulink/Logic and Bit Operations/Bit Set  iBit=4
  Bit Set1 : simulink/Logic and Bit Operations/Bit Set  iBit=3
  Bit Set2 : simulink/Logic and Bit Operations/Bit Set  iBit=3
  Bit Set4 : simulink/Logic and Bit Operations/Bit Set  iBit=7
  Constant1 : Constant  Value=0  OutDataTypeStr=uint8
  Constant7 : Constant  Value=0  OutDataTypeStr=boolean
  Delay2 : Delay  DelayLength=1  InitialCondition=1
  Delay3 : Delay  DelayLength=1  InitialCondition=0
  Logical Operator : Logic  Operator=OR  AllPortsSameDT=off  OutDataTypeStr=boolean
  Switch{1..4} (4 alike) : Switch  Criteria=u2 ~= 0
  Dfc_id : Outport  OutDataTypeStr=uint8
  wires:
  Dfc_id_nv/1 -> Bit Clear2/1, Bit Set4/1, Bit Clear1/1
  Bit Set4/1 -> Bit Set/1
  Constant7/1 -> Delay2/1
  Delay2/1 -> Switch2/2
  Switch3/1 -> Switch2/3
  Bit Clear2/1 -> Switch2/1
  Switch2/1 -> Delay3/1, Switch1/1
  Bit Set1/1 -> Switch3/1
  Bit Set/1 -> Bit Set1/1
  Switch4/1 -> Switch3/3
  Err/1 -> Logical Operator/2, Switch3/2
  Bit Set2/1 -> Switch4/1
  Bit Clear1/1 -> Bit Set2/1
  Delay3/1 -> Switch4/3
  Heal/1 -> Logical Operator/1, Switch4/2
  Logical Operator/1 -> Switch1/2
  Constant1/1 -> Switch1/3
  Switch1/1 -> Dfc_id/1

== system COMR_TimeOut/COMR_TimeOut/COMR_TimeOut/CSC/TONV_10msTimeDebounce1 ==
  note: Turn On Delay Time Deboune
  u : Inport
  T : Inport  Port=2
  Add : Sum
  Constant1 : Constant  Value=0  OutDataTypeStr=single
  Constant2 : Constant  OutDataTypeStr=uint8
  Constant3 : Constant  Value=0  OutDataTypeStr=uint8
  Constant4 : Constant  Value=0.01  OutDataTypeStr=single
  Delay : Delay  DelayLength=1  InitialCondition=0
  MinMax : MinMax  Inputs=2
  Product : Product  OutMin=[0]  OutMax=[65535]  OutDataTypeStr=single
  Relational Operator : RelationalOperator  Operator=>  OutDataTypeStr=boolean  RndMeth=Simplest
  Switch : Switch  Criteria=u2 ~= 0
  Switch1 : Switch  Criteria=u2 ~= 0
  y : Outport
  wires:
  MinMax/1 -> Add/2
  T/1 -> Relational Operator/2, MinMax/1
  Relational Operator/1 -> y/1
  Delay/1 -> MinMax/2
  Switch/1 -> Add/1
  Product/1 -> Delay/1, Relational Operator/1
  Add/1 -> Product/2
  Constant1/1 -> Switch/3
  Constant4/1 -> Switch/1
  u/1 -> Switch/2, Switch1/2
  Constant2/1 -> Switch1/1
  Constant3/1 -> Switch1/3
  Switch1/1 -> Product/1

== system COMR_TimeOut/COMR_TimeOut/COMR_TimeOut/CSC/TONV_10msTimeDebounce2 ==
  note: Turn On Delay Time Deboune
  u : Inport
  T : Inport  Port=2
  Add : Sum
  Constant1 : Constant  Value=0  OutDataTypeStr=single
  Constant2 : Constant  OutDataTypeStr=uint8
  Constant3 : Constant  Value=0  OutDataTypeStr=uint8
  Constant4 : Constant  Value=0.01  OutDataTypeStr=single
  Delay : Delay  DelayLength=1  InitialCondition=0
  MinMax : MinMax  Inputs=2
  Product : Product  OutMin=[0]  OutMax=[65535]  OutDataTypeStr=single
  Relational Operator : RelationalOperator  Operator=>  OutDataTypeStr=boolean  RndMeth=Simplest
  Switch : Switch  Criteria=u2 ~= 0
  Switch1 : Switch  Criteria=u2 ~= 0
  y : Outport
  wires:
  MinMax/1 -> Add/2
  T/1 -> Relational Operator/2, MinMax/1
  Relational Operator/1 -> y/1
  Delay/1 -> MinMax/2
  Switch/1 -> Add/1
  Product/1 -> Delay/1, Relational Operator/1
  Add/1 -> Product/2
  Constant1/1 -> Switch/3
  Constant4/1 -> Switch/1
  u/1 -> Switch/2, Switch1/2
  Constant2/1 -> Switch1/1
  Constant3/1 -> Switch1/3
  Switch1/1 -> Product/1

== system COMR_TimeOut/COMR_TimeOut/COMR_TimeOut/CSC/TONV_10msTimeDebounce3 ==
  note: Turn On Delay Time Deboune
  u : Inport
  T : Inport  Port=2
  Add : Sum
  Constant1 : Constant  Value=0  OutDataTypeStr=single
  Constant2 : Constant  OutDataTypeStr=uint8
  Constant3 : Constant  Value=0  OutDataTypeStr=uint8
  Constant4 : Constant  Value=0.01  OutDataTypeStr=single
  Delay : Delay  DelayLength=1  InitialCondition=0
  MinMax : MinMax  Inputs=2
  Product : Product  OutMin=[0]  OutMax=[65535]  OutDataTypeStr=single
  Relational Operator : RelationalOperator  Operator=>  OutDataTypeStr=boolean  RndMeth=Simplest
  Switch : Switch  Criteria=u2 ~= 0
  Switch1 : Switch  Criteria=u2 ~= 0
  y : Outport
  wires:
  MinMax/1 -> Add/2
  T/1 -> Relational Operator/2, MinMax/1
  Relational Operator/1 -> y/1
  Delay/1 -> MinMax/2
  Switch/1 -> Add/1
  Product/1 -> Delay/1, Relational Operator/1
  Add/1 -> Product/2
  Constant1/1 -> Switch/3
  Constant4/1 -> Switch/1
  u/1 -> Switch/2, Switch1/2
  Constant2/1 -> Switch1/1
  Constant3/1 -> Switch1/3
  Switch1/1 -> Product/1

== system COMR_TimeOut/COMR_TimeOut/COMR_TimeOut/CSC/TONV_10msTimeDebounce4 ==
  note: Turn On Delay Time Deboune
  u : Inport
  T : Inport  Port=2
  Add : Sum
  Constant1 : Constant  Value=0  OutDataTypeStr=single
  Constant2 : Constant  OutDataTypeStr=uint8
  Constant3 : Constant  Value=0  OutDataTypeStr=uint8
  Constant4 : Constant  Value=0.01  OutDataTypeStr=single
  Delay : Delay  DelayLength=1  InitialCondition=0
  MinMax : MinMax  Inputs=2
  Product : Product  OutMin=[0]  OutMax=[65535]  OutDataTypeStr=single
  Relational Operator : RelationalOperator  Operator=>  OutDataTypeStr=boolean  RndMeth=Simplest
  Switch : Switch  Criteria=u2 ~= 0
  Switch1 : Switch  Criteria=u2 ~= 0
  y : Outport
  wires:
  MinMax/1 -> Add/2
  T/1 -> Relational Operator/2, MinMax/1
  Relational Operator/1 -> y/1
  Delay/1 -> MinMax/2
  Switch/1 -> Add/1
  Product/1 -> Delay/1, Relational Operator/1
  Add/1 -> Product/2
  Constant1/1 -> Switch/3
  Constant4/1 -> Switch/1
  u/1 -> Switch/2, Switch1/2
  Constant2/1 -> Switch1/1
  Constant3/1 -> Switch1/3
  Switch1/1 -> Product/1

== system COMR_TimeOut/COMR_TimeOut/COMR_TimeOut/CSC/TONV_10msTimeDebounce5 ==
  note: Turn On Delay Time Deboune
  u : Inport
  T : Inport  Port=2
  Add : Sum
  Constant1 : Constant  Value=0  OutDataTypeStr=single
  Constant2 : Constant  OutDataTypeStr=uint8
  Constant3 : Constant  Value=0  OutDataTypeStr=uint8
  Constant4 : Constant  Value=0.01  OutDataTypeStr=single
  Delay : Delay  DelayLength=1  InitialCondition=0
  MinMax : MinMax  Inputs=2
  Product : Product  OutMin=[0]  OutMax=[65535]  OutDataTypeStr=single
  Relational Operator : RelationalOperator  Operator=>  OutDataTypeStr=boolean  RndMeth=Simplest
  Switch : Switch  Criteria=u2 ~= 0
  Switch1 : Switch  Criteria=u2 ~= 0
  y : Outport
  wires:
  Switch1/1 -> Product/1
  Constant3/1 -> Switch1/3
  Constant2/1 -> Switch1/1
  u/1 -> Switch1/2, Switch/2
  Constant4/1 -> Switch/1
  Constant1/1 -> Switch/3
  Add/1 -> Product/2
  Product/1 -> Relational Operator/1, Delay/1
  Switch/1 -> Add/1
  Delay/1 -> MinMax/2
  Relational Operator/1 -> y/1
  T/1 -> MinMax/1, Relational Operator/2
  MinMax/1 -> Add/2

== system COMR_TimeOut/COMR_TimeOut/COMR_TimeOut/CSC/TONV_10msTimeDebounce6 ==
  note: Turn On Delay Time Deboune
  u : Inport
  T : Inport  Port=2
  Add : Sum
  Constant1 : Constant  Value=0  OutDataTypeStr=single
  Constant2 : Constant  OutDataTypeStr=uint8
  Constant3 : Constant  Value=0  OutDataTypeStr=uint8
  Constant4 : Constant  Value=0.01  OutDataTypeStr=single
  Delay : Delay  DelayLength=1  InitialCondition=0
  MinMax : MinMax  Inputs=2
  Product : Product  OutMin=[0]  OutMax=[65535]  OutDataTypeStr=single
  Relational Operator : RelationalOperator  Operator=>  OutDataTypeStr=boolean  RndMeth=Simplest
  Switch : Switch  Criteria=u2 ~= 0
  Switch1 : Switch  Criteria=u2 ~= 0
  y : Outport
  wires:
  MinMax/1 -> Add/2
  T/1 -> Relational Operator/2, MinMax/1
  Relational Operator/1 -> y/1
  Delay/1 -> MinMax/2
  Switch/1 -> Add/1
  Product/1 -> Delay/1, Relational Operator/1
  Add/1 -> Product/2
  Constant1/1 -> Switch/3
  Constant4/1 -> Switch/1
  u/1 -> Switch/2, Switch1/2
  Constant2/1 -> Switch1/1
  Constant3/1 -> Switch1/3
  Switch1/1 -> Product/1

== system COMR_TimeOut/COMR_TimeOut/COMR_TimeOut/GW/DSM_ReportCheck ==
  note: Fault report to diagnostic management system
  Dfc_id_nv : Inport  OutDataTypeStr=uint8
  Err : Inport  Port=2
  Heal : Inport  Port=3
  Bit Clear1 : simulink/Logic and Bit Operations/Bit Clear  iBit=4
  Bit Clear2 : simulink/Logic and Bit Operations/Bit Clear  iBit=3
  Bit Set : simulink/Logic and Bit Operations/Bit Set  iBit=4
  Bit Set1 : simulink/Logic and Bit Operations/Bit Set  iBit=3
  Bit Set2 : simulink/Logic and Bit Operations/Bit Set  iBit=3
  Bit Set4 : simulink/Logic and Bit Operations/Bit Set  iBit=7
  Constant1 : Constant  Value=0  OutDataTypeStr=uint8
  Constant7 : Constant  Value=0  OutDataTypeStr=boolean
  Delay2 : Delay  DelayLength=1  InitialCondition=1
  Delay3 : Delay  DelayLength=1  InitialCondition=0
  Logical Operator : Logic  Operator=OR  AllPortsSameDT=off  OutDataTypeStr=boolean
  Switch{1..4} (4 alike) : Switch  Criteria=u2 ~= 0
  Dfc_id : Outport  OutDataTypeStr=uint8
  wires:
  Dfc_id_nv/1 -> Bit Clear2/1, Bit Set4/1, Bit Clear1/1
  Bit Set4/1 -> Bit Set/1
  Constant7/1 -> Delay2/1
  Delay2/1 -> Switch2/2
  Switch3/1 -> Switch2/3
  Bit Clear2/1 -> Switch2/1
  Switch2/1 -> Delay3/1, Switch1/1
  Bit Set1/1 -> Switch3/1
  Bit Set/1 -> Bit Set1/1
  Switch4/1 -> Switch3/3
  Err/1 -> Logical Operator/2, Switch3/2
  Bit Set2/1 -> Switch4/1
  Bit Clear1/1 -> Bit Set2/1
  Delay3/1 -> Switch4/3
  Heal/1 -> Logical Operator/1, Switch4/2
  Logical Operator/1 -> Switch1/2
  Constant1/1 -> Switch1/3
  Switch1/1 -> Dfc_id/1

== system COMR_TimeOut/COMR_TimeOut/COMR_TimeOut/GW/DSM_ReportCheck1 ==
  note: Fault report to diagnostic management system
  Dfc_id_nv : Inport  OutDataTypeStr=uint8
  Err : Inport  Port=2
  Heal : Inport  Port=3
  Bit Clear1 : simulink/Logic and Bit Operations/Bit Clear  iBit=4
  Bit Clear2 : simulink/Logic and Bit Operations/Bit Clear  iBit=3
  Bit Set : simulink/Logic and Bit Operations/Bit Set  iBit=4
  Bit Set1 : simulink/Logic and Bit Operations/Bit Set  iBit=3
  Bit Set2 : simulink/Logic and Bit Operations/Bit Set  iBit=3
  Bit Set4 : simulink/Logic and Bit Operations/Bit Set  iBit=7
  Constant1 : Constant  Value=0  OutDataTypeStr=uint8
  Constant7 : Constant  Value=0  OutDataTypeStr=boolean
  Delay2 : Delay  DelayLength=1  InitialCondition=1
  Delay3 : Delay  DelayLength=1  InitialCondition=0
  Logical Operator : Logic  Operator=OR  AllPortsSameDT=off  OutDataTypeStr=boolean
  Switch{1..4} (4 alike) : Switch  Criteria=u2 ~= 0
  Dfc_id : Outport  OutDataTypeStr=uint8
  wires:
  Switch1/1 -> Dfc_id/1
  Constant1/1 -> Switch1/3
  Logical Operator/1 -> Switch1/2
  Heal/1 -> Switch4/2, Logical Operator/1
  Delay3/1 -> Switch4/3
  Bit Clear1/1 -> Bit Set2/1
  Bit Set2/1 -> Switch4/1
  Err/1 -> Switch3/2, Logical Operator/2
  Switch4/1 -> Switch3/3
  Bit Set/1 -> Bit Set1/1
  Bit Set1/1 -> Switch3/1
  Switch2/1 -> Switch1/1, Delay3/1
  Bit Clear2/1 -> Switch2/1
  Switch3/1 -> Switch2/3
  Delay2/1 -> Switch2/2
  Constant7/1 -> Delay2/1
  Bit Set4/1 -> Bit Set/1
  Dfc_id_nv/1 -> Bit Clear1/1, Bit Set4/1, Bit Clear2/1

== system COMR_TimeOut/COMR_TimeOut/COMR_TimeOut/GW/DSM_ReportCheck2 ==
  note: Fault report to diagnostic management system
  Dfc_id_nv : Inport  OutDataTypeStr=uint8
  Err : Inport  Port=2
  Heal : Inport  Port=3
  Bit Clear1 : simulink/Logic and Bit Operations/Bit Clear  iBit=4
  Bit Clear2 : simulink/Logic and Bit Operations/Bit Clear  iBit=3
  Bit Set : simulink/Logic and Bit Operations/Bit Set  iBit=4
  Bit Set1 : simulink/Logic and Bit Operations/Bit Set  iBit=3
  Bit Set2 : simulink/Logic and Bit Operations/Bit Set  iBit=3
  Bit Set4 : simulink/Logic and Bit Operations/Bit Set  iBit=7
  Constant1 : Constant  Value=0  OutDataTypeStr=uint8
  Constant7 : Constant  Value=0  OutDataTypeStr=boolean
  Delay2 : Delay  DelayLength=1  InitialCondition=1
  Delay3 : Delay  DelayLength=1  InitialCondition=0
  Logical Operator : Logic  Operator=OR  AllPortsSameDT=off  OutDataTypeStr=boolean
  Switch{1..4} (4 alike) : Switch  Criteria=u2 ~= 0
  Dfc_id : Outport  OutDataTypeStr=uint8
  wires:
  Dfc_id_nv/1 -> Bit Clear2/1, Bit Set4/1, Bit Clear1/1
  Bit Set4/1 -> Bit Set/1
  Constant7/1 -> Delay2/1
  Delay2/1 -> Switch2/2
  Switch3/1 -> Switch2/3
  Bit Clear2/1 -> Switch2/1
  Switch2/1 -> Delay3/1, Switch1/1
  Bit Set1/1 -> Switch3/1
  Bit Set/1 -> Bit Set1/1
  Switch4/1 -> Switch3/3
  Err/1 -> Logical Operator/2, Switch3/2
  Bit Set2/1 -> Switch4/1
  Bit Clear1/1 -> Bit Set2/1
  Delay3/1 -> Switch4/3
  Heal/1 -> Logical Operator/1, Switch4/2
  Logical Operator/1 -> Switch1/2
  Constant1/1 -> Switch1/3
  Switch1/1 -> Dfc_id/1

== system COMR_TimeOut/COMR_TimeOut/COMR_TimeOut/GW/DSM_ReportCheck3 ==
  note: Fault report to diagnostic management system
  Dfc_id_nv : Inport  OutDataTypeStr=uint8
  Err : Inport  Port=2
  Heal : Inport  Port=3
  Bit Clear1 : simulink/Logic and Bit Operations/Bit Clear  iBit=4
  Bit Clear2 : simulink/Logic and Bit Operations/Bit Clear  iBit=3
  Bit Set : simulink/Logic and Bit Operations/Bit Set  iBit=4
  Bit Set1 : simulink/Logic and Bit Operations/Bit Set  iBit=3
  Bit Set2 : simulink/Logic and Bit Operations/Bit Set  iBit=3
  Bit Set4 : simulink/Logic and Bit Operations/Bit Set  iBit=7
  Constant1 : Constant  Value=0  OutDataTypeStr=uint8
  Constant7 : Constant  Value=0  OutDataTypeStr=boolean
  Delay2 : Delay  DelayLength=1  InitialCondition=1
  Delay3 : Delay  DelayLength=1  InitialCondition=0
  Logical Operator : Logic  Operator=OR  AllPortsSameDT=off  OutDataTypeStr=boolean
  Switch{1..4} (4 alike) : Switch  Criteria=u2 ~= 0
  Dfc_id : Outport  OutDataTypeStr=uint8
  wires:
  Switch1/1 -> Dfc_id/1
  Constant1/1 -> Switch1/3
  Logical Operator/1 -> Switch1/2
  Heal/1 -> Switch4/2, Logical Operator/1
  Delay3/1 -> Switch4/3
  Bit Clear1/1 -> Bit Set2/1
  Bit Set2/1 -> Switch4/1
  Err/1 -> Switch3/2, Logical Operator/2
  Switch4/1 -> Switch3/3
  Bit Set/1 -> Bit Set1/1
  Bit Set1/1 -> Switch3/1
  Switch2/1 -> Switch1/1, Delay3/1
  Bit Clear2/1 -> Switch2/1
  Switch3/1 -> Switch2/3
  Delay2/1 -> Switch2/2
  Constant7/1 -> Delay2/1
  Bit Set4/1 -> Bit Set/1
  Dfc_id_nv/1 -> Bit Clear1/1, Bit Set4/1, Bit Clear2/1

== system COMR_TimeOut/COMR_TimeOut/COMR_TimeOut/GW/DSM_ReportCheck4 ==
  note: Fault report to diagnostic management system
  Dfc_id_nv : Inport  OutDataTypeStr=uint8
  Err : Inport  Port=2
  Heal : Inport  Port=3
  Bit Clear1 : simulink/Logic and Bit Operations/Bit Clear  iBit=4
  Bit Clear2 : simulink/Logic and Bit Operations/Bit Clear  iBit=3
  Bit Set : simulink/Logic and Bit Operations/Bit Set  iBit=4
  Bit Set1 : simulink/Logic and Bit Operations/Bit Set  iBit=3
  Bit Set2 : simulink/Logic and Bit Operations/Bit Set  iBit=3
  Bit Set4 : simulink/Logic and Bit Operations/Bit Set  iBit=7
  Constant1 : Constant  Value=0  OutDataTypeStr=uint8
  Constant7 : Constant  Value=0  OutDataTypeStr=boolean
  Delay2 : Delay  DelayLength=1  InitialCondition=1
  Delay3 : Delay  DelayLength=1  InitialCondition=0
  Logical Operator : Logic  Operator=OR  AllPortsSameDT=off  OutDataTypeStr=boolean
  Switch{1..4} (4 alike) : Switch  Criteria=u2 ~= 0
  Dfc_id : Outport  OutDataTypeStr=uint8
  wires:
  Dfc_id_nv/1 -> Bit Clear2/1, Bit Set4/1, Bit Clear1/1
  Bit Set4/1 -> Bit Set/1
  Constant7/1 -> Delay2/1
  Delay2/1 -> Switch2/2
  Switch3/1 -> Switch2/3
  Bit Clear2/1 -> Switch2/1
  Switch2/1 -> Delay3/1, Switch1/1
  Bit Set1/1 -> Switch3/1
  Bit Set/1 -> Bit Set1/1
  Switch4/1 -> Switch3/3
  Err/1 -> Logical Operator/2, Switch3/2
  Bit Set2/1 -> Switch4/1
  Bit Clear1/1 -> Bit Set2/1
  Delay3/1 -> Switch4/3
  Heal/1 -> Logical Operator/1, Switch4/2
  Logical Operator/1 -> Switch1/2
  Constant1/1 -> Switch1/3
  Switch1/1 -> Dfc_id/1

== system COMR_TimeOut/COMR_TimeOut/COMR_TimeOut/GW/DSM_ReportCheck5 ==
  note: Fault report to diagnostic management system
  Dfc_id_nv : Inport  OutDataTypeStr=uint8
  Err : Inport  Port=2
  Heal : Inport  Port=3
  Bit Clear1 : simulink/Logic and Bit Operations/Bit Clear  iBit=4
  Bit Clear2 : simulink/Logic and Bit Operations/Bit Clear  iBit=3
  Bit Set : simulink/Logic and Bit Operations/Bit Set  iBit=4
  Bit Set1 : simulink/Logic and Bit Operations/Bit Set  iBit=3
  Bit Set2 : simulink/Logic and Bit Operations/Bit Set  iBit=3
  Bit Set4 : simulink/Logic and Bit Operations/Bit Set  iBit=7
  Constant1 : Constant  Value=0  OutDataTypeStr=uint8
  Constant7 : Constant  Value=0  OutDataTypeStr=boolean
  Delay2 : Delay  DelayLength=1  InitialCondition=1
  Delay3 : Delay  DelayLength=1  InitialCondition=0
  Logical Operator : Logic  Operator=OR  AllPortsSameDT=off  OutDataTypeStr=boolean
  Switch{1..4} (4 alike) : Switch  Criteria=u2 ~= 0
  Dfc_id : Outport  OutDataTypeStr=uint8
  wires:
  Switch1/1 -> Dfc_id/1
  Constant1/1 -> Switch1/3
  Logical Operator/1 -> Switch1/2
  Heal/1 -> Switch4/2, Logical Operator/1
  Delay3/1 -> Switch4/3
  Bit Clear1/1 -> Bit Set2/1
  Bit Set2/1 -> Switch4/1
  Err/1 -> Switch3/2, Logical Operator/2
  Switch4/1 -> Switch3/3
  Bit Set/1 -> Bit Set1/1
  Bit Set1/1 -> Switch3/1
  Switch2/1 -> Switch1/1, Delay3/1
  Bit Clear2/1 -> Switch2/1
  Switch3/1 -> Switch2/3
  Delay2/1 -> Switch2/2
  Constant7/1 -> Delay2/1
  Bit Set4/1 -> Bit Set/1
  Dfc_id_nv/1 -> Bit Clear1/1, Bit Set4/1, Bit Clear2/1

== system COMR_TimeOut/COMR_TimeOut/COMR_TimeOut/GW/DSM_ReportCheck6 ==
  note: Fault report to diagnostic management system
  Dfc_id_nv : Inport  OutDataTypeStr=uint8
  Err : Inport  Port=2
  Heal : Inport  Port=3
  Bit Clear1 : simulink/Logic and Bit Operations/Bit Clear  iBit=4
  Bit Clear2 : simulink/Logic and Bit Operations/Bit Clear  iBit=3
  Bit Set : simulink/Logic and Bit Operations/Bit Set  iBit=4
  Bit Set1 : simulink/Logic and Bit Operations/Bit Set  iBit=3
  Bit Set2 : simulink/Logic and Bit Operations/Bit Set  iBit=3
  Bit Set4 : simulink/Logic and Bit Operations/Bit Set  iBit=7
  Constant1 : Constant  Value=0  OutDataTypeStr=uint8
  Constant7 : Constant  Value=0  OutDataTypeStr=boolean
  Delay2 : Delay  DelayLength=1  InitialCondition=1
  Delay3 : Delay  DelayLength=1  InitialCondition=0
  Logical Operator : Logic  Operator=OR  AllPortsSameDT=off  OutDataTypeStr=boolean
  Switch{1..4} (4 alike) : Switch  Criteria=u2 ~= 0
  Dfc_id : Outport  OutDataTypeStr=uint8
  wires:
  Dfc_id_nv/1 -> Bit Clear2/1, Bit Set4/1, Bit Clear1/1
  Bit Set4/1 -> Bit Set/1
  Constant7/1 -> Delay2/1
  Delay2/1 -> Switch2/2
  Switch3/1 -> Switch2/3
  Bit Clear2/1 -> Switch2/1
  Switch2/1 -> Delay3/1, Switch1/1
  Bit Set1/1 -> Switch3/1
  Bit Set/1 -> Bit Set1/1
  Switch4/1 -> Switch3/3
  Err/1 -> Logical Operator/2, Switch3/2
  Bit Set2/1 -> Switch4/1
  Bit Clear1/1 -> Bit Set2/1
  Delay3/1 -> Switch4/3
  Heal/1 -> Logical Operator/1, Switch4/2
  Logical Operator/1 -> Switch1/2
  Constant1/1 -> Switch1/3
  Switch1/1 -> Dfc_id/1
